(* Logix 5000 AddOnInstructionDefinition export SPEL_Above; software revision 30.01; part 9 of 9 *)

ADD_ON_INSTRUCTION SPEL_XYLimSet   (* revision 1.0, vendor SEIKO EPSON CORP. *)
// Sets the allowable motion area by specifying the
// lower and upper limit positions.
VAR_OUTPUT
   InCycle : BOOL; {access Read Only, visible}
   Done : BOOL; {access Read Only, visible}
   Error : BOOL; {access Read Only, visible}
END_VAR
VAR_INPUT
   Start : BOOL; {required}
   XLower : REAL; {access Read Only, required}
   XUpper : REAL; {access Read Only, required}
   YLower : REAL; {access Read Only, required}
   YUpper : REAL; {access Read Only, required}
   ZLower : REAL; {access Read Only, required}
   ZUpper : REAL; {access Read Only, required}
END_VAR
VAR_IN_OUT
   ExtInputs : AB:ETHERNET_MODULE_INT_128Bytes:I:0; {required}
   ExtOutputs : AB:ETHERNET_MODULE_INT_128Bytes:O:0; {required}
END_VAR
VAR_OUTPUT
   ErrCode1 : INT; {access Read Only, visible}
   ErrCode2 : INT; {access Read Only, visible}
END_VAR
VAR
   ExecXYLimSetZ : SPEL_ExecCmd := (MaxTime := 3000); {access None}
   ExecXYLimSetY : SPEL_ExecCmd := (MaxTime := 3000); {access None}
   ExecXYLimSetX : SPEL_ExecCmd := (MaxTime := 3000); {access None}
   upperLimit_INTS : INT[2]; {access None}
   StartInit : BOOL[32]; {access None}
   OneShotStart : BOOL[32]; {access None}
   lowerLimit_INTS : INT[2]; {access None}
   Lowerx1000 : DINT; {access None}
   Upperx1000 : DINT; {access None}
   ExecTimeout : DINT; {access None}
END_VAR

ROUTINE Logic   (* ladder *)
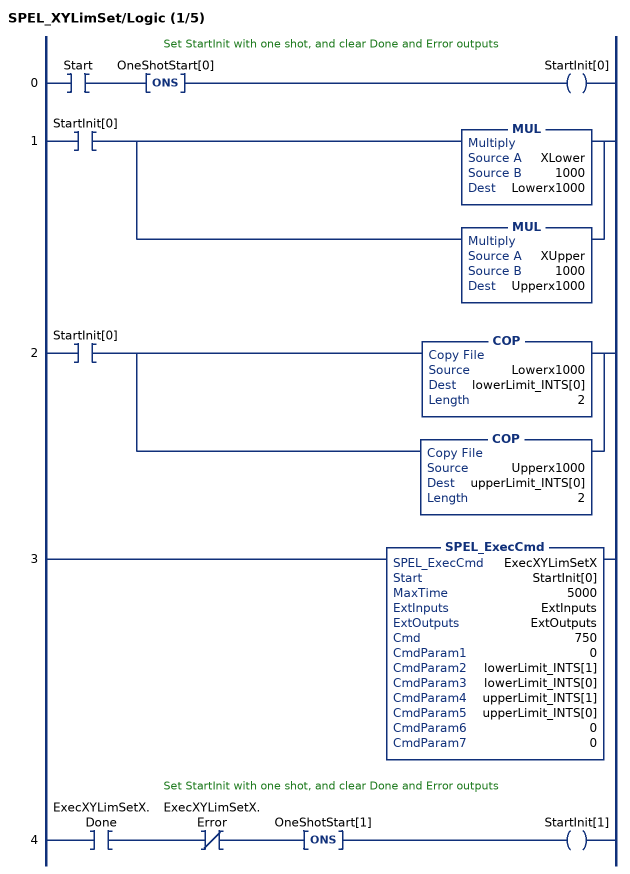
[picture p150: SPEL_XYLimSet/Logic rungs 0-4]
   // Set StartInit with one shot, and clear Done and Error outputs
   0: XIC(Start)ONS(OneShotStart[0])OTE(StartInit[0]);
   1: XIC(StartInit[0])[MUL(XLower,1000,Lowerx1000) ,MUL(XUpper,1000,Upperx1000) ];
   2: XIC(StartInit[0])[COP(Lowerx1000,lowerLimit_INTS[0],2) ,COP(Upperx1000,upperLimit_INTS[0],2) ];
   3: SPEL_ExecCmd(ExecXYLimSetX,StartInit[0],5000,ExtInputs,ExtOutputs,750,0,lowerLimit_INTS[1],lowerLimit_INTS[0],upperLimit_INTS[1],upperLimit_INTS[0],0,0);
   // Set StartInit with one shot, and clear Done and Error outputs
   4: XIC(ExecXYLimSetX.Done)XIO(ExecXYLimSetX.Error)ONS(OneShotStart[1])OTE(StartInit[1]);
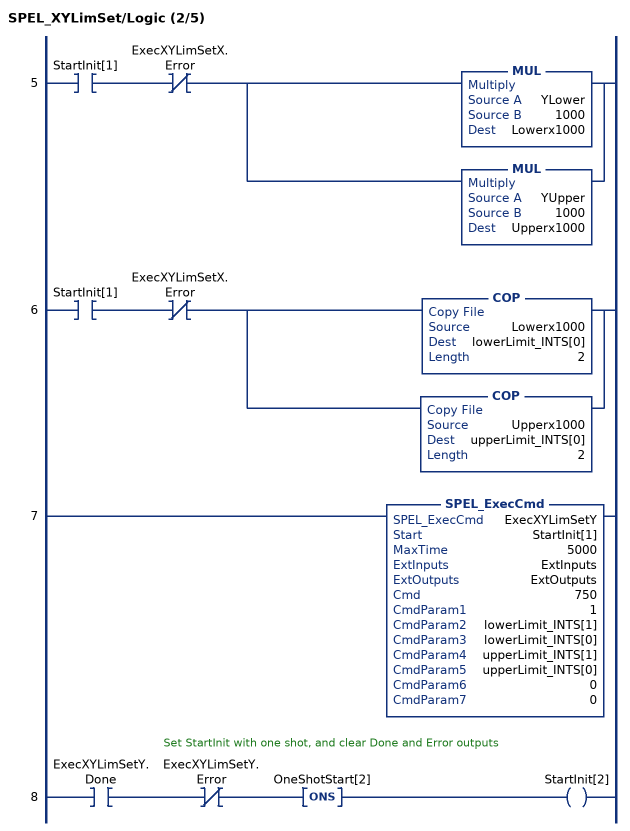
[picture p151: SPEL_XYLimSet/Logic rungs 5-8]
   5: XIC(StartInit[1])XIO(ExecXYLimSetX.Error)[MUL(YLower,1000,Lowerx1000) ,MUL(YUpper,1000,Upperx1000) ];
   6: XIC(StartInit[1])XIO(ExecXYLimSetX.Error)[COP(Lowerx1000,lowerLimit_INTS[0],2) ,COP(Upperx1000,upperLimit_INTS[0],2) ];
   7: SPEL_ExecCmd(ExecXYLimSetY,StartInit[1],5000,ExtInputs,ExtOutputs,750,1,lowerLimit_INTS[1],lowerLimit_INTS[0],upperLimit_INTS[1],upperLimit_INTS[0],0,0);
   // Set StartInit with one shot, and clear Done and Error outputs
   8: XIC(ExecXYLimSetY.Done)XIO(ExecXYLimSetY.Error)ONS(OneShotStart[2])OTE(StartInit[2]);
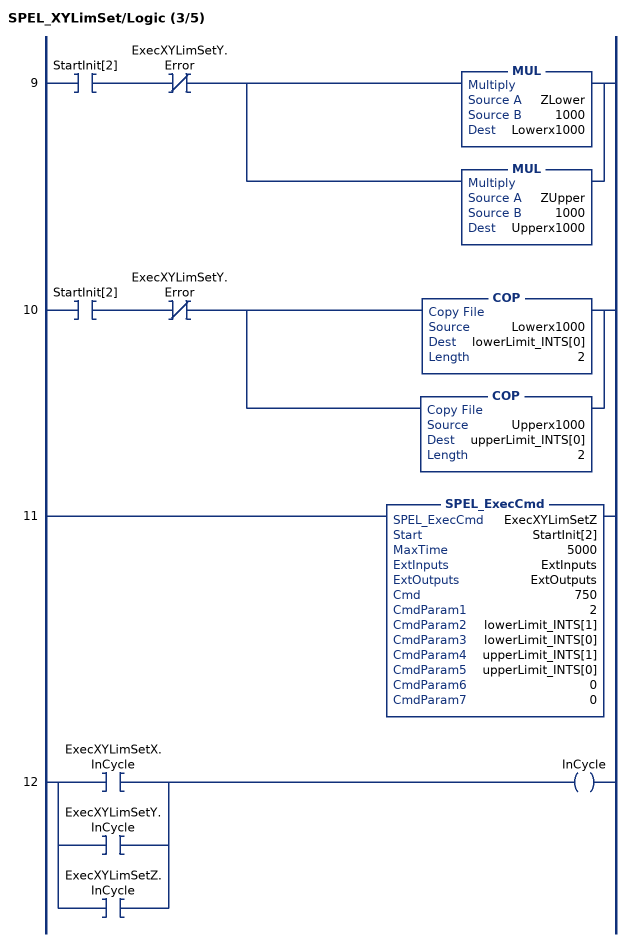
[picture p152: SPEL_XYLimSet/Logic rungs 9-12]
   9: XIC(StartInit[2])XIO(ExecXYLimSetY.Error)[MUL(ZLower,1000,Lowerx1000) ,MUL(ZUpper,1000,Upperx1000) ];
   10: XIC(StartInit[2])XIO(ExecXYLimSetY.Error)[COP(Lowerx1000,lowerLimit_INTS[0],2) ,COP(Upperx1000,upperLimit_INTS[0],2) ];
   11: SPEL_ExecCmd(ExecXYLimSetZ,StartInit[2],5000,ExtInputs,ExtOutputs,750,2,lowerLimit_INTS[1],lowerLimit_INTS[0],upperLimit_INTS[1],upperLimit_INTS[0],0,0);
   12: [XIC(ExecXYLimSetX.InCycle) ,XIC(ExecXYLimSetY.InCycle) ,XIC(ExecXYLimSetZ.InCycle) ]OTE(InCycle);
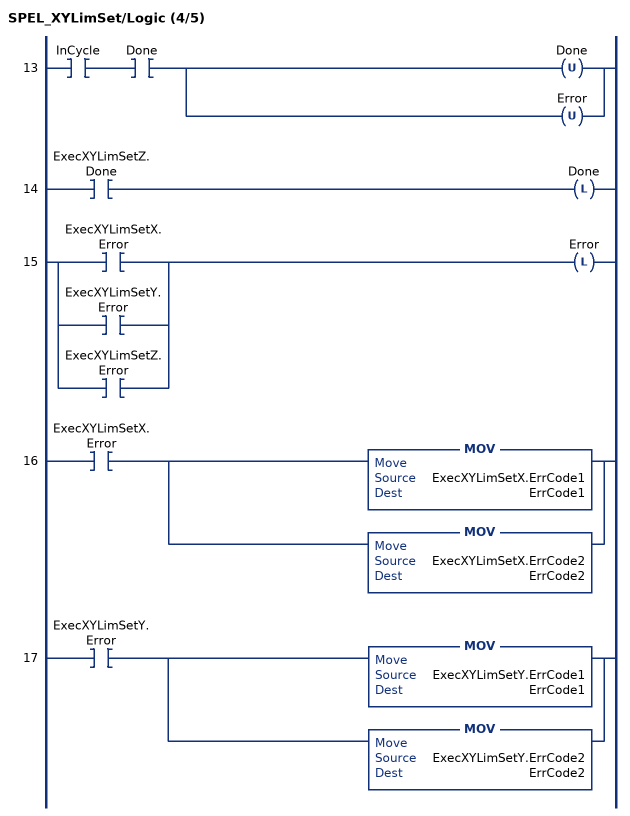
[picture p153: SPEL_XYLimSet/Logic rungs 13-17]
   13: XIC(InCycle)XIC(Done)[OTU(Done) ,OTU(Error) ];
   14: XIC(ExecXYLimSetZ.Done)OTL(Done);
   15: [XIC(ExecXYLimSetX.Error) ,XIC(ExecXYLimSetY.Error) ,XIC(ExecXYLimSetZ.Error) ]OTL(Error);
   16: XIC(ExecXYLimSetX.Error)[MOV(ExecXYLimSetX.ErrCode1,ErrCode1) ,MOV(ExecXYLimSetX.ErrCode2,ErrCode2) ];
   17: XIC(ExecXYLimSetY.Error)[MOV(ExecXYLimSetY.ErrCode1,ErrCode1) ,MOV(ExecXYLimSetY.ErrCode2,ErrCode2) ];
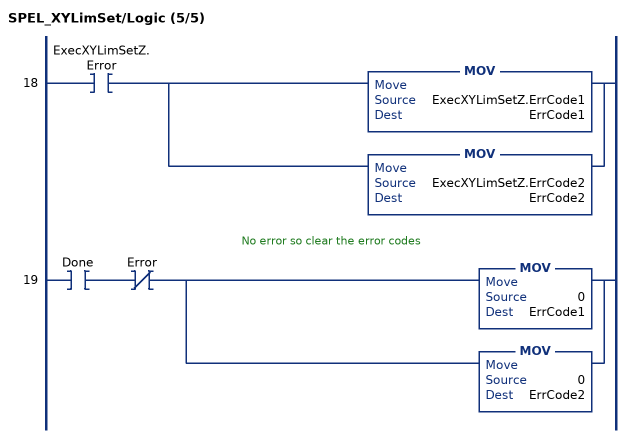
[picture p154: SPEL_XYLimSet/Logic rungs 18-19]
   18: XIC(ExecXYLimSetZ.Error)[MOV(ExecXYLimSetZ.ErrCode1,ErrCode1) ,MOV(ExecXYLimSetZ.ErrCode2,ErrCode2) ];
   // No error so clear the error codes
   19: XIC(Done)XIO(Error)[MOV(0,ErrCode1) ,MOV(0,ErrCode2) ];
END_ROUTINE
END_ADD_ON_INSTRUCTION
